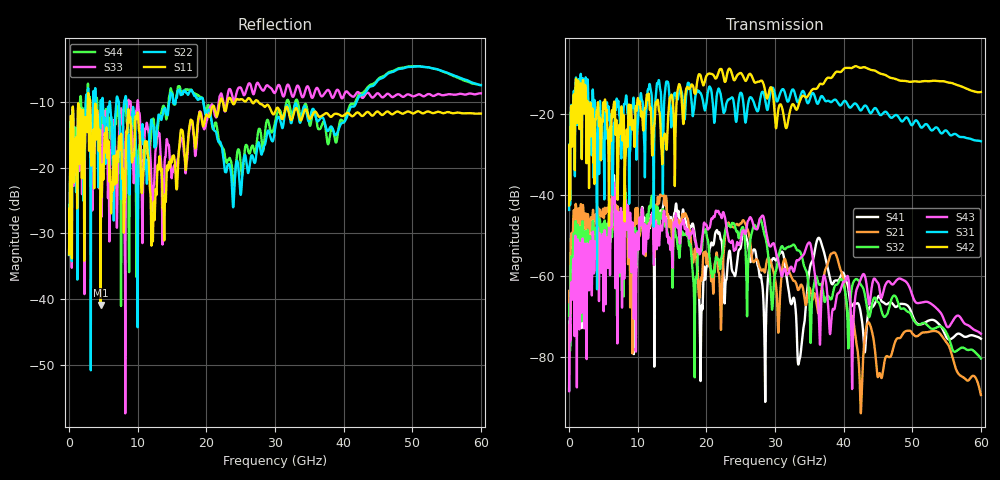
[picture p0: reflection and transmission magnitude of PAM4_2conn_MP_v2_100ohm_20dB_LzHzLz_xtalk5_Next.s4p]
! Info: Touchstone file created by Circ.  Input file=FAB50GbE_2conn_Midplane_Examax_Topo2_v2_100ohm_20dB_LzHzLz.circ
# Hz S RI R 50
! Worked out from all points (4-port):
!   6000 points, 10 MHz to 60 GHz, reference 50 ohm
!   strongest paths, dB at 10 MHz, 15.01 GHz, 30.01 GHz, 45.01 GHz, 60 GHz:
!     S42: -42.6, -15.7, -21.2, -9.7, -14.6
!     S31: -43.7, -20.3, -15.2, -19.5, -26.8
!     S43: -88.5, -55.3, -53.1, -61.8, -74.4
!     S32: -70.0, -55.1, -59.6, -66.5, -80.5
!     S21: -69.6, -51.4, -60.8, -85.1, -89.5
!     S41: -88.3, -50.3, -56.1, -65.2, -75.6
!   lowest |S11| = -40.9 dB at 4.6 GHz (marker M1), VSWR 1.02, Z = 50.9 + j0.209 ohm
!   |S11| at or under -10 dB: start of sweep to 2.729 GHz; 3.081 GHz to 21.98 GHz (18.89 GHz wide, 151 % of centre); 27.61 GHz to end of sweep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
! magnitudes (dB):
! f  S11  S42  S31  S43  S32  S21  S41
! 10 MHz  -33.2  -42.6  -43.7  -88.5  -70.0  -69.6  -88.3
! 1.2 GHz  -22.1  -17.2  -17.6  -53.4  -49.7  -45.8  -49.0
! 4.6 GHz  -40.9  -30.2  -22.7  -53.4  -49.3  -45.1  -51.4
! 28.11 GHz  -10.3  -11.8  -14.6  -45.2  -47.2  -58.7  -61.8
! 33.56 GHz  -12.4  -17.1  -16.5  -55.9  -53.9  -63.1  -80.8
! 36.47 GHz  -12.2  -12.7  -16.6  -73.5  -62.3  -68.0  -50.7
! 60 GHz  -11.7  -14.6  -26.8  -74.4  -80.5  -89.5  -75.6
